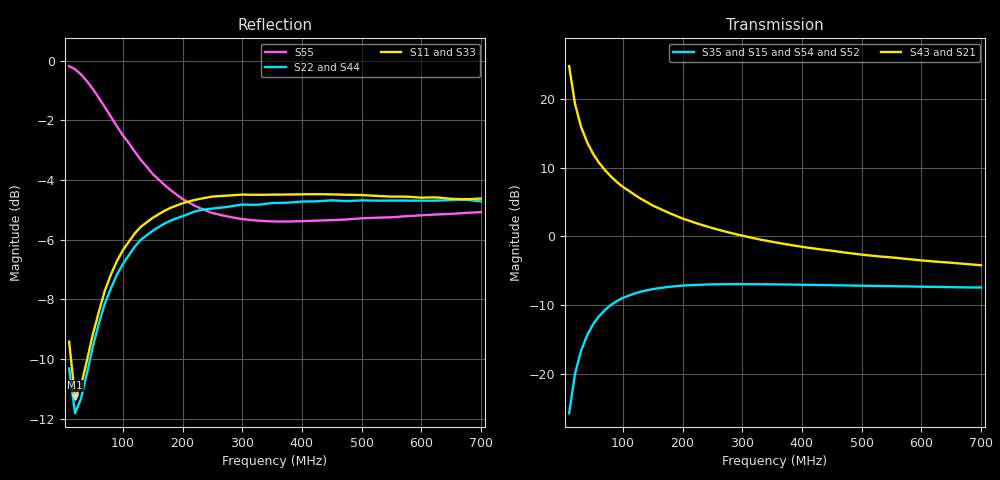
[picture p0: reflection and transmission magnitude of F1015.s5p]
! Date: Mon Aug 07 16:40:39 1995
!  POLYFET RF DEVICES
!  F1015
!  S PARAMETERS
!  VDS=28V, IDQ=800mA
!AWR Design Environment (2053) Wed Feb 04 14:29:15 2004
!freq-unit  param-type  data-format  keyword  impedance-ohms
# MHz  S  MA  R  50
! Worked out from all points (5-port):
!   70 points, 10 MHz to 700 MHz, reference 50 ohm
!   strongest paths, dB at 10 MHz, 180 MHz, 360 MHz, 530 MHz, 700 MHz:
!     S43: 24.8, 3.3, -0.9, -2.9, -4.2
!     S21: 24.8, 3.3, -0.9, -2.9, -4.2
!     S35: -25.8, -7.3, -7.0, -7.2, -7.4
!     S15: -25.8, -7.3, -7.0, -7.2, -7.4
!     S54: -26.1, -7.6, -7.2, -7.3, -7.5
!     S52: -26.1, -7.6, -7.2, -7.3, -7.5
!   lowest |S11| = -11.3 dB at 20 MHz (marker M1), VSWR 1.75, Z = 47.1 - j27.3 ohm
!   |S11| at or under -10 dB: 13.11 MHz to 40.39 MHz (27.27 MHz wide, 102 % of centre)
